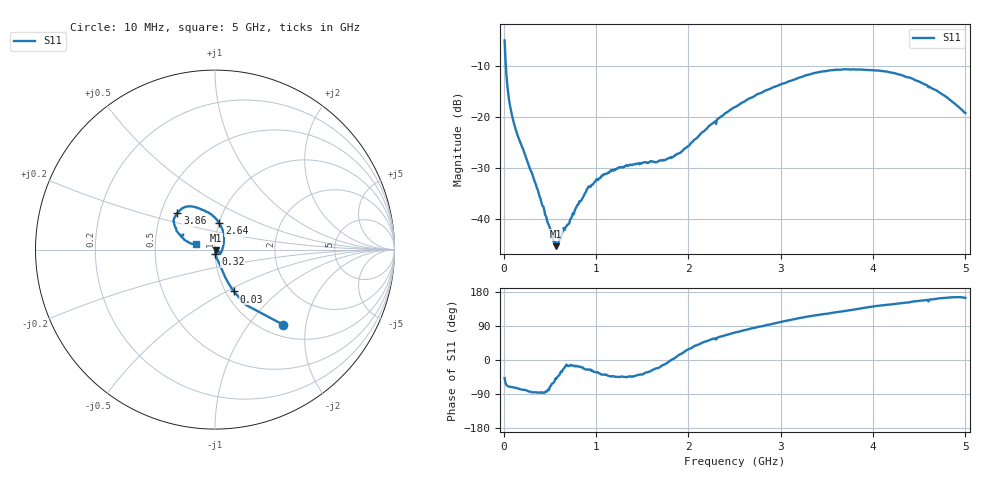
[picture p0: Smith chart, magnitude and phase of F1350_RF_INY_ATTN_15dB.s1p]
! S-parameters for RF_INY input IDT F1350 DPD Demodulator
! Date Measured:  2015-11-25  RGG
!  Port 1 = Pin 3 = RF_INY
! STATE: RF_INY selected, 15 dB attenuation (Gain = Gmax - 15 dB)
! RF Frequency:  10 MHz to 5000 MHz
! RF_INX, IF_I+, IF_I-, IF_Q+, and IF_Q- terminated
! 2300 MHz, 0 dBm signal applied to LO_IN
! Vcc = +5.00 Volts  Icc = approx 275 mA
! NOTES:  The device was measured on a custom printed circuit evaluation board with individual 50 ohm
!  microstrip lines to the RF and LO pins. The 50 ohm microstrip lines were de-embedded using reference
!  plane extensions
! Instrument Manufacturer:  Agilent Technologies
! Instrument Model:  E5071C
! Instrument Serial Number:  MY46419053
! Instrument Firmware Rev:  A.11.31
# HZ  S  RI R 50.00
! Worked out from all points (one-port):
!   500 points, 10 MHz to 5 GHz, reference 50 ohm
!   lowest |S11| = -45.3 dB at 570 MHz (marker M1), VSWR 1.01, Z = 50.4 - j0.416 ohm
!   |S11| at or under -10 dB: 23.44 MHz to end of sweep
!   S11 on the Smith chart (normalised r, x): 10 MHz: 1.22, -1.49; 30 MHz: 1.09, -0.55; 320 MHz: 1.00, -0.05; 2.64 GHz: 1.01, +0.30; 3.86 GHz: 0.61, +0.27; 5 GHz: 0.81, +0.05
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1e7  0.3789 -0.4182
3e7  0.1047 -0.2334
4e7  0.0751 -0.188
6e7  0.0488 -0.1358
8e7  0.0367 -0.1088
1.1e8  0.0266 -0.0835
1.6e8  0.0159 -0.0608
3.2e8  0.00218 -0.0258
5.3e8  0.00326 -0.00607
5.7e8  0.00353 -0.00413
6e8  0.00483 -0.00411
6.4e8  0.00694 -0.00336
9.2e8  0.0189 -0.00907
1.08e9  0.0211 -0.0167
1.26e9  0.0228 -0.0227
1.66e9  0.0336 -0.0135
1.89e9  0.0431 0.00904
2.24e9  0.0495 0.0678
2.51e9  0.0371 0.1205
2.64e9  0.0249 0.1465
3.13e9  -0.0678 0.2205
3.43e9  -0.1383 0.2413
3.76e9  -0.1953 0.2191
3.86e9  -0.2095 0.2047
4.14e9  -0.2307 0.1592
4.38e9  -0.2159 0.1163
4.7e9  -0.1712 0.0551
5e9  -0.1054 0.0307
